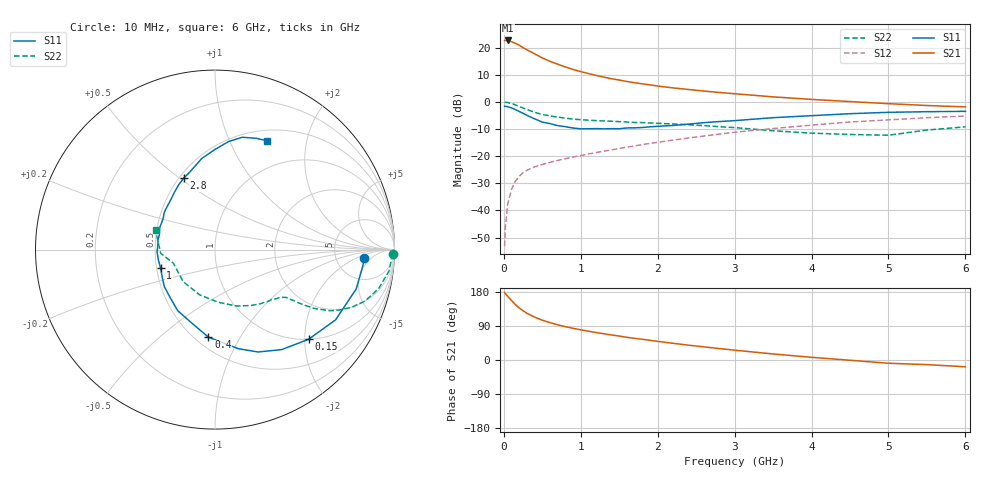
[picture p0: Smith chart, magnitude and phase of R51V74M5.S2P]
! SIEMENS Small Signal Semiconductors
! BFR183
! Si NPN RF Bipolar Junction Transistor in SOT23
! VCE = 1.75 V  IC = 4.5 mA
! Common Emitter S-Parameters:  May  1996
# GHz  S  MA  R  50
!  f  S11  S21  S12  S22
! GHz  MAG  ANG  MAG  ANG  MAG  ANG  MAG  ANG
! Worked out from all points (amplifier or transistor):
!   36 points, 10 MHz to 6 GHz, reference 50 ohm
!   highest |S21| = 22.7 dB at 50 MHz (marker M1)
!   |S21| within 3 dB of that: start of sweep to 272.7 MHz
!   unconditionally stable (mu >= 1): 1.039 GHz to 2.681 GHz
!   at 250 MHz: K = 0.39, MSG = 23.1 dB, |S12| = -26.1 dB
!   at 1.4 GHz: K = 1.07, MAG = 11.6 dB, |S12| = -17.7 dB
!   at 6 GHz: K = 0.90, MSG = 1.7 dB, |S12| = -5.2 dB
!   S11 on the Smith chart (normalised r, x): 10 MHz: 10, -3; 150 MHz: 1.00, -2.09; 400 MHz: 0.58, -0.74; 1 GHz: 0.53, -0.12; 2.8 GHz: 0.53, +0.52; 6 GHz: 0.63, +1.39
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0.01  0.8319 -3.3  13.51 177.8  0.0022 84.7  0.9903 -1.4
0.02  0.8292 -6.1  13.59 175.1  0.005 85.8  0.9857 -2.8
0.05  0.8167 -15.6  13.6 168.0  0.0131 82.7  0.9764 -7.1
0.1  0.7776 -30.2  12.85 157.0  0.0245 74.8  0.9365 -13.5
0.15  0.7221 -43.8  12.06 146.0  0.0349 68.3  0.884 -18.9
0.2  0.6696 -56.3  11.11 137.3  0.0424 64.0  0.8262 -22.9
0.25  0.6189 -67.2  10.03 129.8  0.0496 60.2  0.7725 -25.8
0.3  0.567 -76.8  9.156 123.3  0.0552 57.9  0.726 -28.0
0.4  0.4894 -94.3  7.696 113.3  0.0638 54.5  0.6456 -30.6
0.5  0.4257 -108.7  6.461 105.0  0.0704 53.4  0.5886 -31.8
0.6  0.3989 -121.3  5.613 98.6  0.0773 52.9  0.5529 -32.5
0.7  0.3665 -132.8  4.962 92.9  0.0836 53.4  0.5251 -32.9
0.8  0.35 -143.8  4.41 87.9  0.0899 53.6  0.5024 -33.4
1  0.3199 -161.4  3.621 79.6  0.1027 54.9  0.4716 -34.3
1.1  0.3205 -169.1  3.338 76.1  0.1099 55.6  0.462 -35.2
1.6  0.3318 158.4  2.383 59.9  0.1467 56.7  0.4265 -40.5
2.2  0.369 132.5  1.817 44.1  0.1984 55.4  0.3936 -50.1
2.8  0.4353 113.5  1.497 30.2  0.2558 51.4  0.3503 -63.3
3.5  0.5133 98.2  1.241 15.9  0.3242 44.0  0.2945 -86.1
4.5  0.6078 82.7  1.017 -0.7  0.4273 31.9  0.2516 -134.7
5.5  0.6613 69.7  0.86 -12.2  0.5125 19.2  0.3035 -176.1
6  0.6718 64.5  0.811 -17.9  0.5515 11.0  0.3479 162.1
